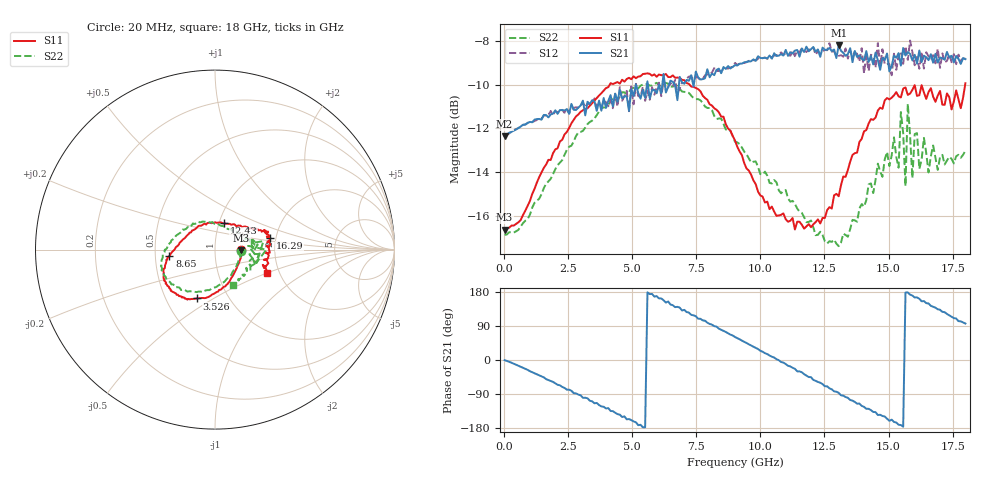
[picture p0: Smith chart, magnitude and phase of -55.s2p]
!Agilent Technologies,N5230A,US43500223,A.07.50.48
!Agilent N5230A: A.07.50.48
!Date: Monday, January 11, 2016 18:30:00
!Correction: S11(Full 2 Port(1,2))
!S21(Full 2 Port(1,2))
!S12(Full 2 Port(1,2))
!S22(Full 2 Port(1,2))
!S2P File: Measurements: S11, S21, S12, S22:
# Hz S  dB  R 50
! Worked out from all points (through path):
!   201 points, 20 MHz to 18 GHz, reference 50 ohm
!   highest |S21| = -8.21 dB at 13.06 GHz (marker M1); lowest = -12.4 dB at 20 MHz (marker M2)
!   group delay of S21, straight-line fit = 97.5 ps
!   lowest |S11| = -16.6 dB at 20 MHz (marker M3), VSWR 1.35, Z = 67.3 - j0.62 ohm
!   |S11| at or under -10 dB: start of sweep to 4.123 GHz; 7.236 GHz to 17.99 GHz (10.76 GHz wide, 85.3 % of centre)
!   |S22| runs from -17.4 to -9.9 dB; largest |S21 - S12| = 0.053
!   S11 on the Smith chart (normalised r, x): 20 MHz: 1.35, -0.01; 3.526 GHz: 0.71, -0.42; 8.65 GHz: 0.59, -0.05; 12.43 GHz: 1.06, +0.32; 16.29 GHz: 1.87, +0.27; 18 GHz: 1.73, -0.50
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2e7  -16.64 -1.8  -12.37 -0.4  -12.34 -0.2  -16.87 -2.1
1.5483e9  -13.81 -69.9  -11.39 -45.8  -11.41 -46.2  -14.73 -72.1
3.0766e9  -11.17 -101.9  -10.73 -99.8  -10.81 -98.4  -12.11 -109.7
3.5261e9  -10.73 -110.6  -10.77 -114.2  -10.63 -112.9  -11.55 -118.4
6.0433e9  -9.54 -142.6  -10.01 162.6  -9.91 160.3  -10.02 -154.5
7.3019e9  -10.09 -155.6  -9.57 119.2  -9.63 117.8  -10.51 -170.1
8.6504e9  -11.81 -171.8  -9.28 74.0  -9.24 72.2  -12.05 170.5
9.01e9  -12.55 -177.7  -9.11 60.7  -9.01 59.7  -12.61 164.3
1.05383e10  -15.80 138.2  -8.57 6.4  -8.68 4.7  -14.36 130.4
1.20666e10  -16.38 82.9  -8.28 -52.5  -8.30 -52.4  -16.53 93.8
1.24262e10  -16.10 70.3  -8.31 -63.5  -8.50 -64.0  -16.87 82.5
1.30555e10  -15.10 47.8  -8.21 -86.7  -8.69 -89.2  -17.39 58.9
1.43141e10  -11.58 25.4  -8.69 -132.3  -8.63 -129.2  -14.52 19.7
1.50333e10  -10.68 20.0  -9.40 -160.3  -9.06 -162.1  -13.73 8.2
1.53929e10  -10.54 19.4  -8.56 -170.8  -8.66 -167.7  -13.80 10.0
1.54828e10  -10.59 18.3  -9.13 -171.6  -8.49 -174.9  -11.25 10.0
1.56626e10  -10.13 18.8  -8.67 177.9  -8.25 178.2  -14.64 6.5
1.57525e10  -10.47 16.8  -8.52 178.5  -8.87 171.9  -10.88 -0.1
1.59323e10  -10.24 16.0  -8.89 170.1  -8.53 165.0  -14.27 -7.7
1.60222e10  -10.02 13.0  -8.63 164.9  -9.12 167.1  -12.26 -5.7
1.62919e10  -10.03 11.8  -8.97 154.9  -8.58 156.3  -13.43 -13.2
1.8e10  -9.94 -23.8  -8.84 96.3  -8.82 91.4  -13.02 -62.6
